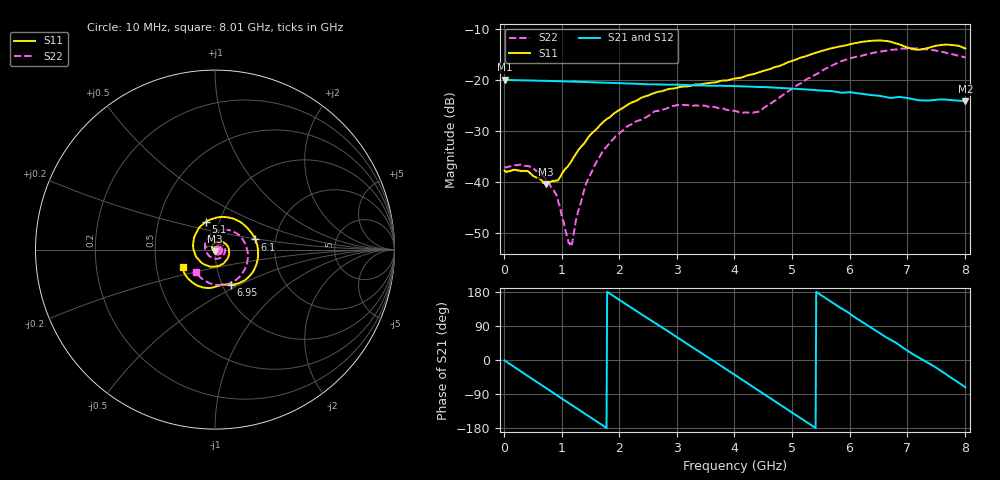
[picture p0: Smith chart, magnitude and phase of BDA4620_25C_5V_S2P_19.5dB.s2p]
!Agilent Technologies,E5071B,MY42404982,A.09.10
!Date: Wed May 06 09:02:29 2026
!Data & Calibration Information:
!Freq	S11:SOLT2(ON)	S21:SOLT2(ON)	S12:SOLT2(ON)	S22:SOLT2(ON)
# Hz S RI R 50
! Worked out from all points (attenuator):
!   801 points, 10 MHz to 8.01 GHz, reference 50 ohm
!   highest |S21| = -19.92 dB at 10 MHz (marker M1); lowest = -24.2 dB at 8.01 GHz (marker M2)
!   lowest |S11| = -40.4 dB at 720 MHz (marker M3), VSWR 1.02, Z = 49.9 - j0.948 ohm
!   |S11| at or under -10 dB: start of sweep to end of sweep
!   |S22| runs from -52.6 to -13.7 dB; largest |S21 - S12| = 0.00044
!   S11 on the Smith chart (normalised r, x): 10 MHz: 1.03, -0.00; 5.1 GHz: 0.86, +0.27; 6.1 GHz: 1.57, +0.19; 6.95 GHz: 1.10, -0.45; 8.01 GHz: 0.68, -0.14
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1e7  0.013 -0.000849  0.101 -0.0021  0.1011 -0.00221  0.014 -0.000494
4.4e8  0.00878 -0.00886  0.0704 -0.0702  0.0705 -0.0704  0.0133 -0.00527
7.2e8  -0.000831 -0.0095  0.0285 -0.0944  0.0285 -0.0946  0.00809 -0.00737
9.2e8  -0.00855 -0.00589  -0.00559 -0.0977  -0.0057 -0.0978  0.00315 -0.0064
1.14e9  -0.0146 0.00364  -0.0417 -0.0877  -0.0417 -0.0879  -0.00199 -0.00157
1.19e9  -0.0154 0.00674  -0.049 -0.0835  -0.0491 -0.0836  -0.00266 0.000104
1.35e9  -0.0156 0.0163  -0.0698 -0.0663  -0.0699 -0.0664  -0.00433 0.00523
1.54e9  -0.0109 0.0287  -0.0867 -0.0398  -0.0869 -0.0398  -0.00393 0.0128
1.77e9  0.00207 0.0408  -0.0945 -0.00296  -0.0947 -0.00295  0.000647 0.0219
2.15e9  0.0361 0.0447  -0.0753 0.0548  -0.0754 0.0549  0.018 0.0306
2.68e9  0.0769 0.00476  -0.00316 0.0909  -0.00303 0.0911  0.0464 0.0192
3.07e9  0.0715 -0.048  0.0537 0.0724  0.0539 0.0724  0.0569 -0.008
4.01e9  -0.0701 -0.0765  0.0672 -0.0559  0.0673 -0.056  -0.0129 -0.0483
4.42e9  -0.1194 -0.00143  0.0141 -0.0846  0.014 -0.0847  -0.0477 -0.0126
5.1e9  -0.0519 0.1536  -0.0702 -0.0427  -0.0704 -0.0426  -0.0194 0.0881
5.35e9  0.019 0.1803  -0.0798 -0.00891  -0.0799 -0.00902  0.0239 0.1059
6.1e9  0.2246 0.0564  -0.028 0.0696  -0.0281 0.0697  0.1639 0.0415
6.68e9  0.1774 -0.1622  0.0377 0.0558  0.0378 0.0561  0.1728 -0.0942
6.95e9  0.0889 -0.1957  0.0585 0.0339  0.0586 0.0339  0.1354 -0.1534
7.2e9  0.0359 -0.1958  0.0633 0.00739  0.0634 0.0074  0.0761 -0.1895
7.59e9  -0.0721 -0.2094  0.0567 -0.0316  0.0567 -0.0316  -0.0246 -0.1892
8.01e9  -0.181 -0.0954  0.0193 -0.0588  0.0193 -0.0588  -0.1079 -0.1266
